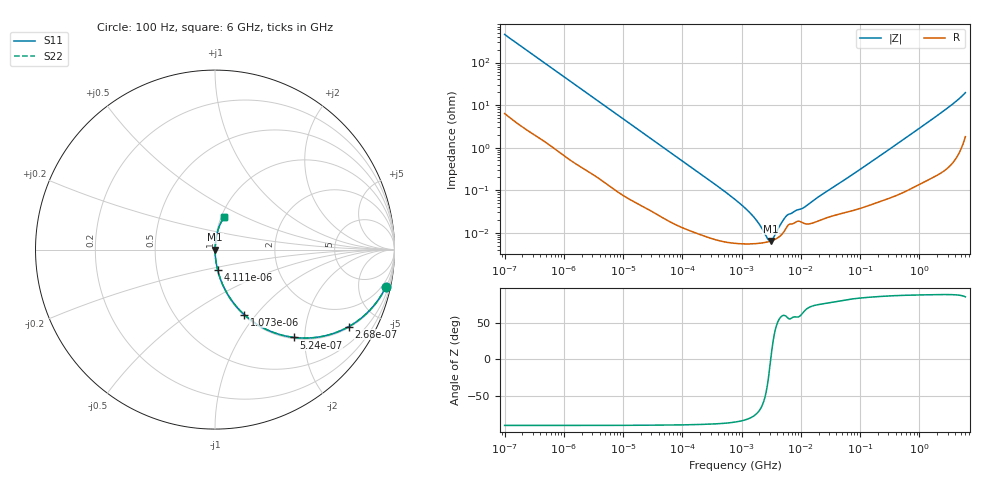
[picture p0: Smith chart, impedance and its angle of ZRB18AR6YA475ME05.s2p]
!Murata Part Number: ZRB18AR6YA475ME05
!These Parameters are Measured in Series Mode Connection
!Data Generated on Jun 10, 2025
!  o--ll--o
!Port1  Port2
!  o------o
!Operation Temp=25[degC], DC Bias Voltage=0[V]
!Freq. Start=100[Hz] Stop=6[GHz] 401[Steps]
# Hz S RI R 50
!Freq.(Hz) S11(Real) S11(Imag) S21(Real) S21(Imag) S12(Real) S12(Imag) S22(Real) S22(Imag)
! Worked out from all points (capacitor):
!   401 points, 100 Hz to 6 GHz, reference 50 ohm
!   read as one part in series: C = 3.47 uF near 109 Hz
!   lowest |Z| = 6.37 mohm at 3.104 MHz (marker M1)
!   series resonance near 3.101 MHz, so ESL is about 760 pH
!   S11 on the Smith chart (normalised r, x): 100 Hz: 1.13, -9.14; 268 Hz: 1.05, -3.44; 524 Hz: 1.03, -1.77; 1.073 kHz: 1.01, -0.87; 4.111 kHz: 1.00, -0.23; 6 GHz: 1.04, +0.39
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100  0.9517 -0.2075  0.0483 0.2075  0.0483 0.2075  0.9517 -0.2075
164  0.8841 -0.3136  0.1159 0.3136  0.1159 0.3136  0.8841 -0.3136
268  0.7447 -0.4293  0.2553 0.4293  0.2553 0.4293  0.7447 -0.4293
524  0.4399 -0.4893  0.5601 0.4893  0.5601 0.4893  0.4399 -0.4893
1073  0.1625 -0.3621  0.8375 0.3621  0.8375 0.3621  0.1625 -0.3621
2008  0.0546 -0.2201  0.9454 0.2201  0.9454 0.2201  0.0546 -0.2201
4111  0.0148 -0.113  0.9852 0.113  0.9852 0.113  0.0148 -0.113
10527  0.00276 -0.0451  0.9972 0.0451  0.9972 0.0451  0.00276 -0.0451
40335  0.000396 -0.012  0.9996 0.012  0.9996 0.012  0.000396 -0.012
774597  5.66e-05 -0.000603  0.9999 0.000603  0.9999 0.000603  5.66e-05 -0.000603
1449809  5.49e-05 -0.00027  0.9999 0.00027  0.9999 0.00027  5.49e-05 -0.00027
2372521  5.84e-05 -8.81e-05  0.9999 8.81e-05  0.9999 8.81e-05  5.84e-05 -8.81e-05
2594782  5.97e-05 -5.84e-05  0.9999 5.84e-05  0.9999 5.84e-05  5.97e-05 -5.84e-05
3103719  6.37e-05 3e-07  0.9999 -3e-07  0.9999 -3e-07  6.37e-05 3e-07
3882480  7.28e-05 7.51e-05  0.9999 -7.51e-05  0.9999 -7.51e-05  7.28e-05 7.51e-05
5311619  0.000111 0.000189  0.9999 -0.000189  0.9999 -0.000189  0.000111 0.000189
6075234  0.00015 0.000221  0.9999 -0.000221  0.9999 -0.000221  0.00015 0.000221
1.087309e7  0.00017 0.000338  0.9998 -0.000338  0.9998 -0.000338  0.00017 0.000338
1.555665e7  0.000168 0.000522  0.9998 -0.000522  0.9998 -0.000522  0.000168 0.000522
3.124326e8  0.00073 0.00912  0.9993 -0.00912  0.9993 -0.00912  0.00073 0.00912
2.048624e9  0.00559 0.0574  0.9944 -0.0574  0.9944 -0.0574  0.00559 0.0574
6e9  0.0528 0.1821  0.9472 -0.1821  0.9472 -0.1821  0.0528 0.1821
